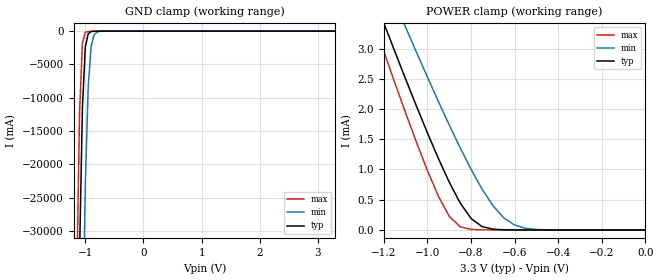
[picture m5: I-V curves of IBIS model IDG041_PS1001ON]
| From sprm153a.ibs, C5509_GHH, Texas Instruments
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| Pin_model   IDG041_PS1001ON
[Model]   IDG041_PS1001ON
 Model_type   Input
 Polarity   Non-Inverting
 Vinl  =  1.08
 Vinh  =  2.10
|Variable   typ   min   max
 C_comp   2.073pF   2.058pF   2.151pF
[Temperature Range]   25   125   -40
[Voltage Range]   3.3   3.0   3.6
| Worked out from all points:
|   GND clamp passes 1 mA (typ) near -0.59 V on its own axis
|   POWER clamp passes 1 mA (typ) near -0.93 V on its own axis
[GND Clamp]
|Voltage   I(typ)   I(min)   I(max)
-3.3V     -2.127kA   -2.167kA   -2.109kA
-1.15V    -66.48A    -117.1A    -39.31A
-1.1V     -33.84A    -80.11A    -12.46A
-1.05V    -11.54A    -47.82A    -1.806A
-1V       -2.382A    -22.98A    -205.2mA
-950mV    -392.2mA   -8.238A    -52.19mA
-900mV    -76.29mA   -2.294A    -31.7mA
-850mV    -25.68mA   -572.4mA   -22.88mA
-800mV    -14.12mA   -143.2mA   -15.79mA
-600mV    -1.143mA   -2.299mA   -876.7uA
3.3V      189.6pA    15.32uA    -31.53uA
[POWER Clamp]
|Voltage   I(typ)   I(min)   I(max)
-3.3V     24.14mA    22.92mA    25.86mA
-1.25V    3.893mA    4.624mA    3.472mA
-1.2V     3.422mA    4.197mA    2.952mA
-1.1V     2.497mA    3.353mA    1.937mA
-1V       1.606mA    2.529mA    983.7uA
-900mV    791.6uA    1.737mA    227.3uA
-850mV    447.6uA    1.361mA    52.71uA
-800mV    190.8uA    1.005mA    9.021uA
-750mV    56.57uA    680.9uA    2.07uA
-650mV    2.655uA    201uA      444.5nA
-500mV    47.83nA    8.483uA    15.08nA
0V        189.6pA    2.741nA    178.5pA
